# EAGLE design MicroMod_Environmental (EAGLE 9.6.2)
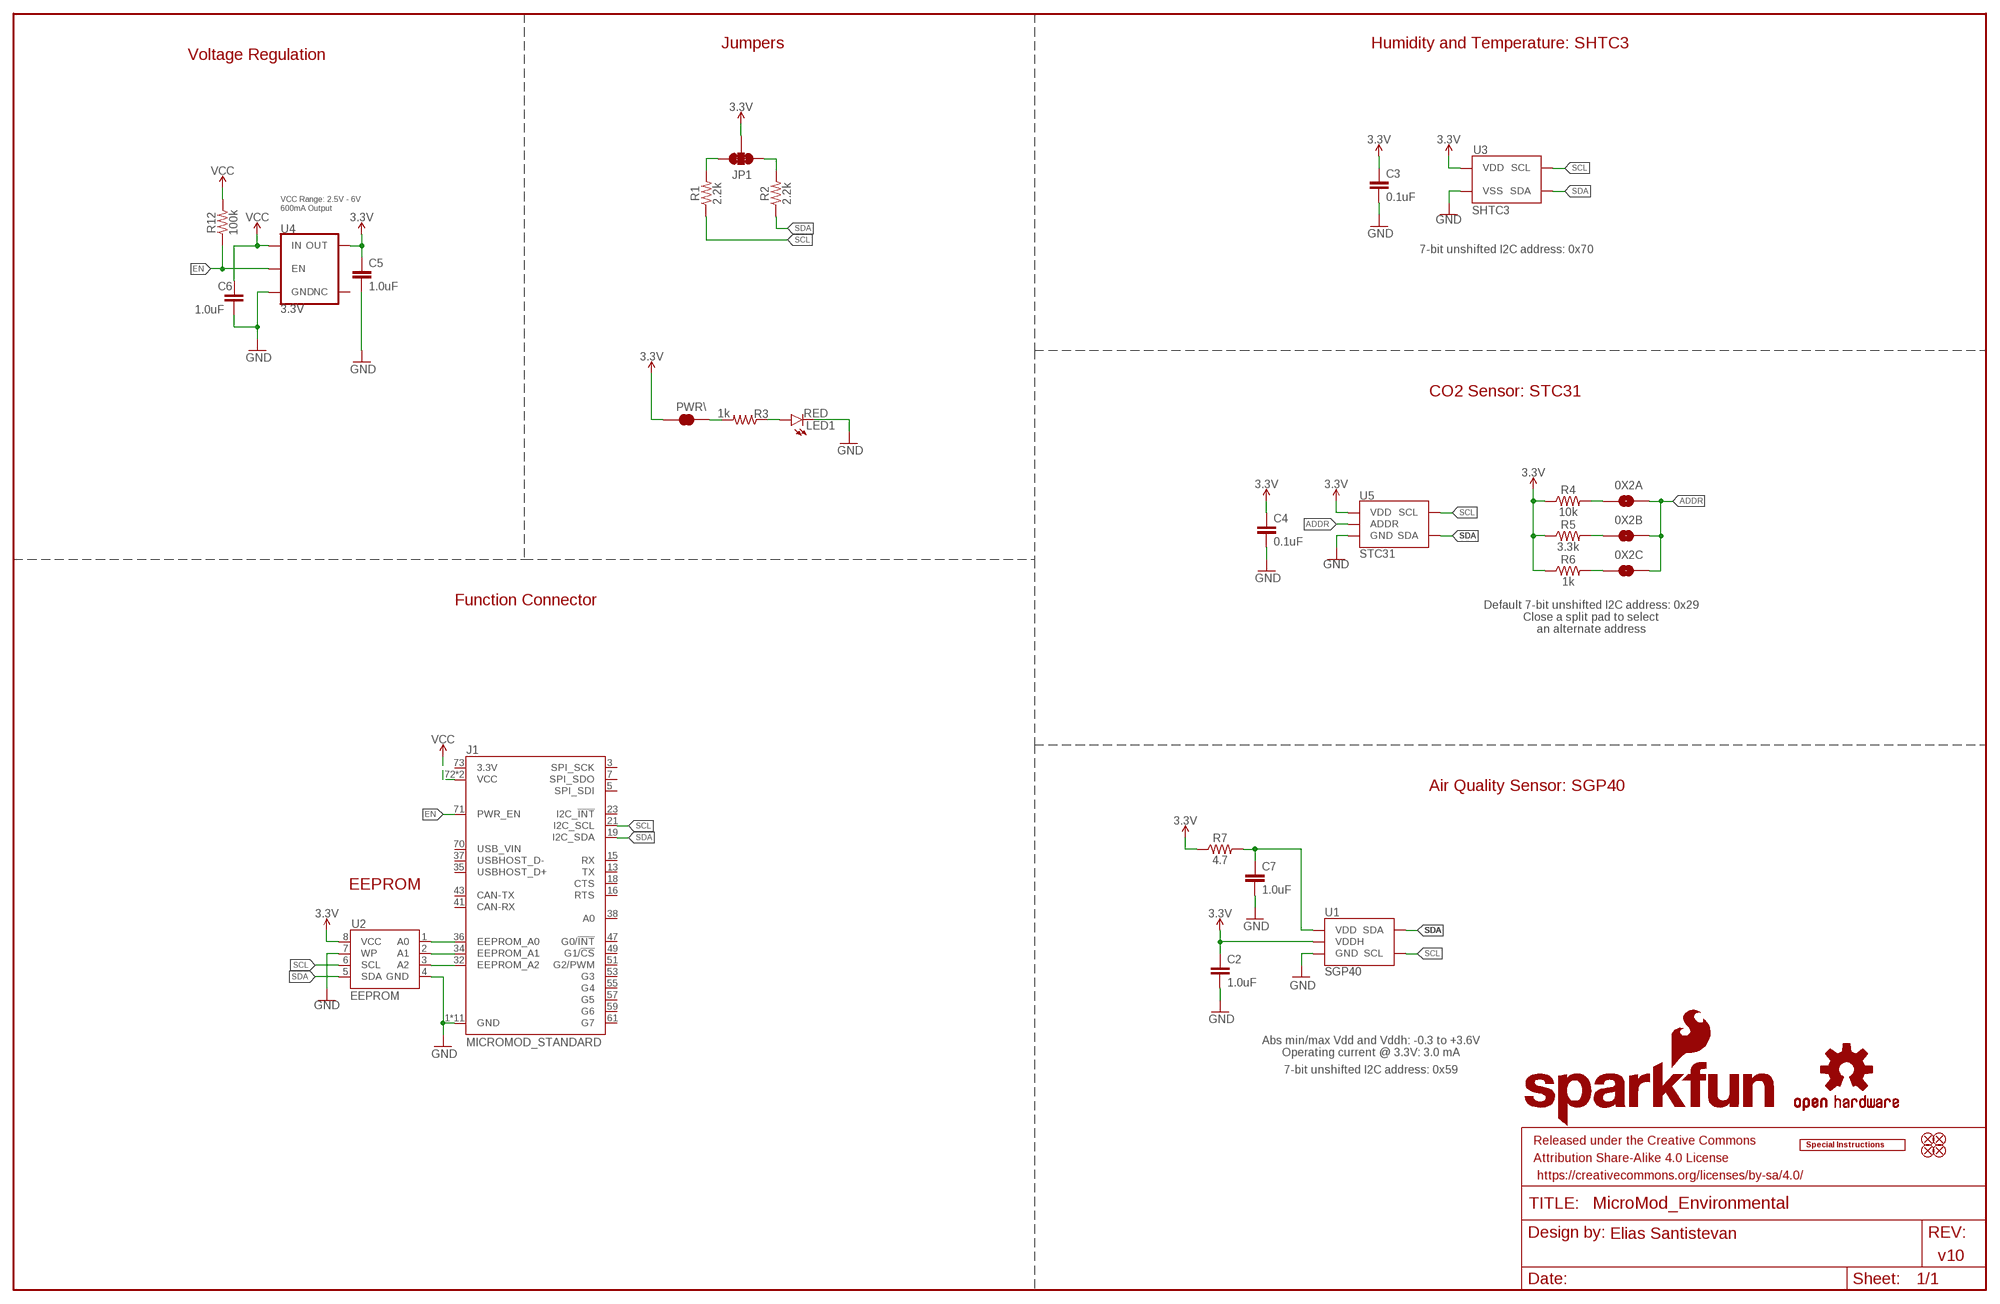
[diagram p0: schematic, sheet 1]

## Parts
0X2A  JUMPER-SMT_2_NO_SILK  [SMT-JUMPER_2_NO_SILK]
0X2B  JUMPER-SMT_2_NO_SILK  [SMT-JUMPER_2_NO_SILK]
0X2C  JUMPER-SMT_2_NO_SILK  [SMT-JUMPER_2_NO_SILK]
C2  1.0uF  1.0UF-0603-16V-10%-X7R  [0603]
C3  0.1uF  0.1UF-0603-25V-5%  [0603]
C4  0.1uF  0.1UF-0603-25V-5%  [0603]
C5  1.0uF  1.0UF-0603-16V-10%  [0603]
C6  1.0uF  1.0UF-0603-16V-10%  [0603]
C7  1.0uF  1.0UF-0603-16V-10%-X7R  [0603]
FD1  FIDUCIAL1X2  [FIDUCIAL-1X2]
FD2  FIDUCIAL1X2  [FIDUCIAL-1X2]
FD3  FIDUCIAL1X2  [FIDUCIAL-1X2]
FD4  FIDUCIAL1X2  [FIDUCIAL-1X2]
FRAME1  FRAME-LEDGER  [CREATIVE_COMMONS]
J1  MICROMOD_STANDARD  [M.2-CARD-E-22_FUNCTION_STANDARD]
JP1  JUMPER-SMT_3_2-NC_TRACE_SILK  [SMT-JUMPER_3_2-NC_TRACE_SILK]
LED1  RED  LED-RED0603  [LED-0603]
LOGO1  SFE_LOGO_NAME_FLAME.2_INCH  [SFE_LOGO_NAME_FLAME_.2]
LOGO2  OSHW-LOGOS  [OSHW-LOGO-S]
LOGO3  SPECIAL_INSTRUCTIONS-ORDERING  [ORDERING_INSTRUCTIONS]
PWR\  JUMPER-SMT_2_NC_TRACE_SILK  [SMT-JUMPER_2_NC_TRACE_SILK]
R1  2.2k  2.2KOHM-0603-1/10W-1%  [0603]
R2  2.2k  2.2KOHM-0603-1/10W-1%  [0603]
R3  1k  1KOHM-0603-1/10W-1%  [0603]
R4  10k  10KOHM-0603-1/10W-1%  [0603]
R5  3.3k  3.3KOHM-0603-1/10W-1%  [0603]
R6  1k  1KOHM-0603-1/10W-1%  [0603]
R7  4.7  4.7OHM-0603-1/10W-1%  [0603]
R12  100k  100KOHM-0603-1/10W-1%  [0603]
U1  SGP40  [SGP40]
U2  EEPROM  EEPROM-I2C512K  [SO08]
U3  SHTC3  [SHTC3]
U4  3.3V  V_REG_AP2112K-3.3V  [SOT23-5]
U5  STC31  [STC31]

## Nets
3.3V [Diff pairs]: C2.1 C3.1 C4.1 C5.1 JP1.2 PWR\.2 R4.1 R5.1 R6.1 R7.1 U1.5(VDDH) U2.8(VCC) U3.1(VDD) U4.5(OUT) U5.6(VDD)
A0: J1.36(EEPROM_A0) U2.1(A0)
A1: J1.34(EEPROM_A1) U2.2(A1)
A2: J1.32(EEPROM_A2) U2.3(A2)
ADDR: 0X2A.2 0X2B.2 0X2C.2 U5.3(ADDR)
EN: J1.71(PWR_EN) R12.1 U4.3(EN)
GND: C2.2 C3.2 C4.2 C5.2 C6.2 C7.2 J1.1(GND) J1.33(GND) J1.39(GND) J1.45(GND) J1.75(GND) J1.GND1(GND) J1.GND2(GND) J1.GND3(GND) J1.GND4(GND) J1.GND5(GND) J1.GND6(GND) LED1.C U1.2(GND) U1.4(GND) U1.DIEPAD(GND) U2.4(GND) U2.7(WP) U3.4(VSS) U3.5(VSS) U4.2(GND) U5.1(GND) U5.5(GND) U5.9(GND) U5.11(GND) U5.DIEPAD(GND)
N$1: PWR\.1 R3.2
N$2: C7.1 R7.2 U1.1(VDD)
N$3: JP1.3 R1.2
N$4: JP1.1 R2.2
N$5: 0X2A.1 R4.2
N$6: 0X2B.1 R5.2
N$7: 0X2C.1 R6.2
N$10: LED1.A R3.1
SCL: J1.21(I2C_SCL) R1.1 U1.6(SCL) U2.6(SCL) U3.2(SCL) U5.4(SCL)
SDA: J1.19(I2C_SDA) R2.1 U1.3(SDA) U2.5(SDA) U3.3(SDA) U5.7(SDA)
VCC: C6.1 J1.72(VCC) J1.74(VCC) R12.2 U4.1(IN)
Unconnected: J1.3(SPI_SCK) J1.5(SPI_SDI) J1.7(SPI_SDO) J1.13(TX) J1.15(RX) J1.16(RTS) J1.18(CTS) J1.23(I2C_!INT!) J1.35(USBHOST_D+) J1.37(USBHOST_D-) J1.38(A0) J1.41(CAN-RX) J1.43(CAN-TX) J1.47(G0/!INT!) J1.49(G1/!CS!) J1.51(G2/PWM) J1.53(G3) J1.55(G4) J1.57(G5) J1.59(G6) J1.61(G7) J1.70(USB_VIN) J1.73(3.3V) U4.4(NC)

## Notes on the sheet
- Jumpers | Humidity and Temperature: SHTC3
- Voltage Regulation
- VCC Range: 2.5V - 6V 
  600mA Output
- 7-bit unshifted I2C address: 0x70
- CO2 Sensor: STC31
- Function Connector
- Default 7-bit unshifted I2C address: 0x29
  Close a split pad to select
  an alternate address
- Air Quality Sensor: SGP40
- EEPROM
- Abs min/max Vdd and Vddh: -0.3 to +3.6V
  Operating current @ 3.3V: 3.0 mA
- 7-bit unshifted I2C address: 0x59
- Elias Santistevan
- v10

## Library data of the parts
0X2A 0X2B 0X2C = SparkFun-Jumpers:JUMPER-SMT_2_NO: Normally open jumper
C2 C7 = SparkFun-Capacitors:1.0UF: 1µF ceramic capacitors; PROD_ID: CAP-13930
C3 C4 = SparkFun-Capacitors:0.1UF: 0.1µF ceramic capacitors; PROD_ID: CAP-08604
C5 C6 = SparkFun-Capacitors:1.0UF: 1µF ceramic capacitors; PROD_ID: CAP-00868
FD1-FD4 = SparkFun-Aesthetics:FIDUCIAL: Fiducial Alignment Points
FRAME1 = SparkFun-Aesthetics:FRAME-LEDGER: Schematic Frame - Ledger
J1 = SparkFun-MicroMod-Function:MICROMOD: MicroMod Connector Description: A card edge connector and mating PCB connector to allow various MicroMod Processor Boards to be coupled with various carrier boards of different capabilities. Based on the M.2 standard.
JP1 = SparkFun-Jumpers:JUMPER-SMT_3_2-NC_TRACE: Normally closed trace jumper (2 of 2 connections) This jumper has a trace between all three pads so they are normally closed (NC). Use a razor knife to open the connection(s). For best results follow the IPC guidelines for cutting traces: Cutout at least 0.063 mm (0.005 in). Remove all loose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
LED1 = SparkFun-LED:LED-RED: Red SMD LED; PROD_ID: DIO-00819
LOGO1 = SparkFun-Aesthetics:SFE_LOGO_NAME_FLAME: SparkFun Font Logo w/ Flame
LOGO2 = SparkFun-Aesthetics:OSHW-LOGO: Open-Source Hardware (OSHW) Logo
LOGO3 = SparkFun-Aesthetics:SPECIAL_INSTRUCTIONS: Special Ordering/Production Instructions Alert
PWR\ = SparkFun-Jumpers:JUMPER-SMT_2_NC_TRACE: Normally closed trace jumper
R1 R2 = SparkFun-Resistors:2.2KOHM: 2.2kΩ resistor; PROD_ID: RES-08272
R3 R6 = SparkFun-Resistors:1KOHM: 1kΩ resistor; PROD_ID: RES-07856
R4 = SparkFun-Resistors:10KOHM: 10kΩ resistor; PROD_ID: RES-00824
R5 = SparkFun-Resistors:3.3KOHM: 3.3kΩ resistor; PROD_ID: RES-07851
R7 = SparkFun-Resistors:4.7OHM: 4.7Ω resistor; PROD_ID: RES-15581
R12 = SparkFun-Resistors:100KOHM: 100kΩ resistor; PROD_ID: RES-07828
U1 = SparkFun-Sensors:SGP40: The SGP40 is a digital gas sensor designed for easy integration into air purifiers or demand-controlled ventilation systems.; DIGIKEY_PART: 1649-SGP40-D-R4CT-ND; PROD_ID: IC-15580
U2 = SparkFun-IC-Memory:EEPROM-I2C: I2C EEPROMs, 24LC256 and others 24LC256 Series 256 kb I2C 2 Wire (32 k x 8 Bit) 2.5 V Serial EEPROM SMD - SOIC-8 Datasheet SparkFun Products SparkFun UDB5 - PIC UAV Development Board (GPS-11703); PROD_ID: IC-14645
U3 = SparkFun-Sensors:SHTC3: Sensirion SHTC3 Humidity Sensor The SHTC3 is a digital humidity and temperature sensor designed especially for battery-driven high-volume consumer electronics applications.; PROD_ID: IC-14840
U4 = SparkFun-IC-Power:V_REG_AP2112: AP2112 - 600mA CMOS LDO Regulator w/ Enable The AP2112 is CMOS process low dropout linear regulator with enable function, the regulator delivers a guaranteed 600mA (min.) continuous load current. Features Output Voltage Accuracy: ±1.5% Output Current: 600mA (Min.) Foldback Short Current Protection: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; PROD_ID: VREG-12457
U5 = SparkFun-Sensors:STC31: STC31 CO2 Sensor Based on Thermal Conductivity; MANU_PART: STC31-R3; PROD_ID: IC-16076

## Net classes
1 Antenna: width 1 mm, clearance 0.3 mm

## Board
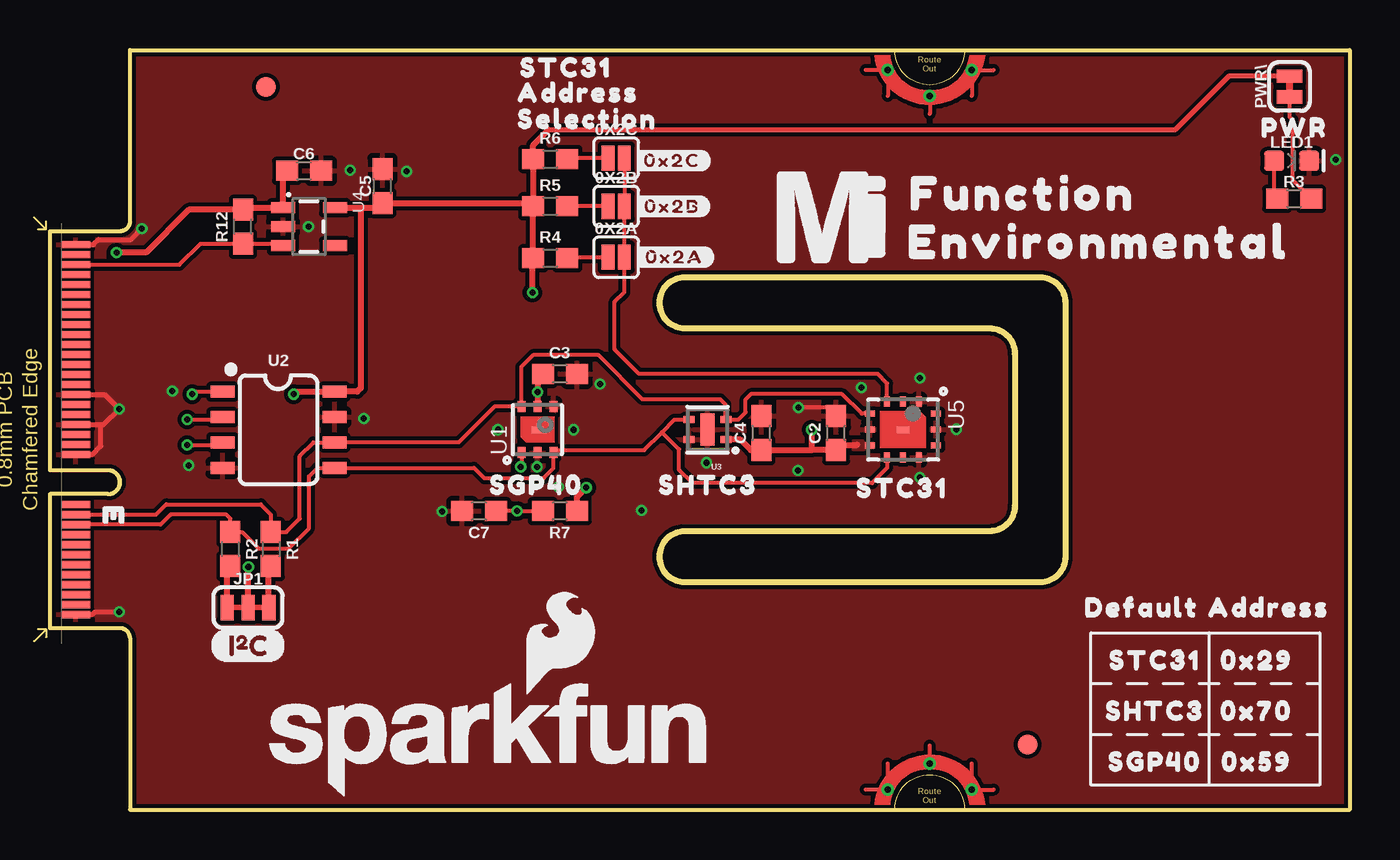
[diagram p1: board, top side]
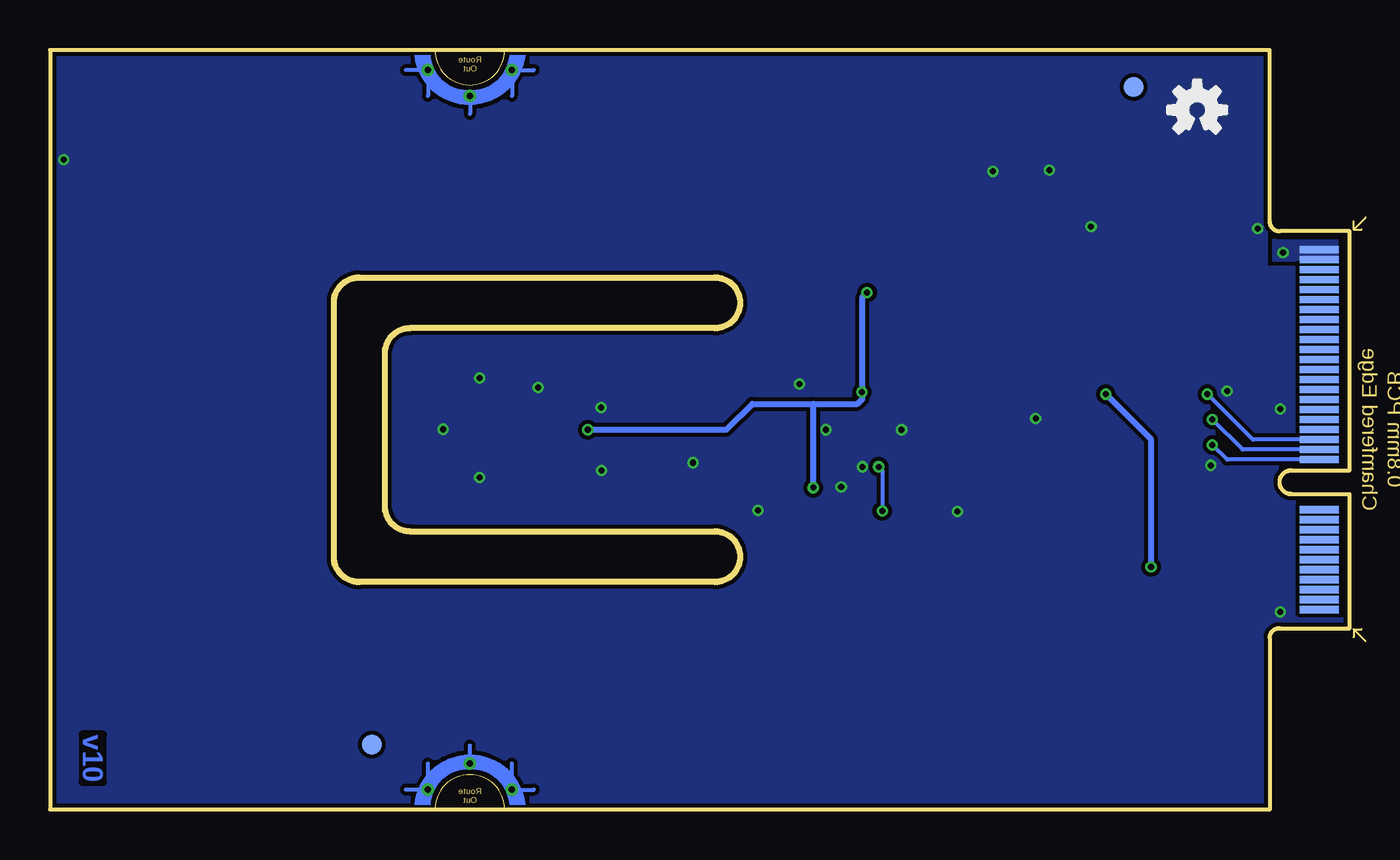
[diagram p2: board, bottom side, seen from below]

Size 65 x 38 mm. Coordinates in mm from the lower left corner, seen from the top.
Outline: 0,9.07 0,15.77 2.9,15.77 arc180 2.9,16.97 0,16.97 0,28.93 3.5,28.93 arc84 4,29.4 4,38 65,38 65,0 4,0 4,8.6 arc85 3.5,9.07 0,9.07
Outline: 30.48,12.65 arc90 31.75,11.38 49.53,11.38 arc90 50.8,12.65 50.8,25.35 arc90 49.53,26.62 31.75,26.62 arc90 30.48,25.35 arc90 31.75,24.08 46.99,24.08 arc-90 48.26,22.81 48.26,15.19 arc-90 46.99,13.92 31.75,13.92 arc90 30.48,12.65
Copper layers (1*16): Top 0.035mm / dielectric 1.5mm / Bottom 0.035mm
Design rules "SparkFun-2-Layer-Minimum-JLCPCB": minimum track width 5mil, minimum drill 0.3mm, track to track 5mil, track to pad 5mil, pad to pad 5mil, via to via 5mil, smd to smd 5mil, copper to edge 7mil, drill to drill 7mil, minimum pad ring 5mil, minimum via ring 5mil, stop-mask expansion 2.5mil, vias tented up to drill 25mil, thermal gap 10mil

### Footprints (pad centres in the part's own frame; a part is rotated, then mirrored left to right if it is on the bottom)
SMT-JUMPER_2_NO_SILK = smd 0.635 x 1.27: 1 -0.406,0; 2 0.406,0
0603 = smd 1.1 x 1: 1 -0.85,0; 2 0.85,0
FIDUCIAL-1X2 = smd 1 x 1: 1 0,0
M.2-CARD-E-22_FUNCTION_STANDARD = smd 0.35 x 1.45: 1 9.25,1.275; 3 8.75,1.275; 5 8.25,1.275; 7 7.75,1.275; 9 7.25,1.275; 11 6.75,1.275; 13 6.25,1.275; 15 5.75,1.275; 17 5.25,1.275; 19 4.75,1.275; 21 4.25,1.275; 23 3.75,1.275; 33 1.25,1.275; 35 0.75,1.275; 37 0.25,1.275; 39 -0.25,1.275; 41 -0.75,1.275; 43 -1.25,1.275; 45 -1.75,1.275; 47 -2.25,1.275; 49 -2.75,1.275; 51 -3.25,1.275; 53 -3.75,1.275; 55 -4.25,1.275; 57 -4.75,1.275; 59 -5.25,1.275; 61 -5.75,1.275; 63 -6.25,1.275; 65 -6.75,1.275; 67 -7.25,1.275; 69 -7.75,1.275; 71 -8.25,1.275; 73 -8.75,1.275; 75 -9.25,1.275 | smd 0.35 x 1.95 bottom: 2 9,1.525; 4 8.5,1.525; 6 8,1.525; 8 7.5,1.525; 10 7,1.525; 12 6.5,1.525; 14 6,1.525; 16 5.5,1.525; 18 5,1.525; 20 4.5,1.525; 22 4,1.525; 32 1.5,1.525; 34 1,1.525; 36 0.5,1.525; 38 0,1.525; 40 -0.5,1.525; 42 -1,1.525; 44 -1.5,1.525; 46 -2,1.525; 48 -2.5,1.525; 50 -3,1.525; 52 -3.5,1.525; 54 -4,1.525; 56 -4.5,1.525; 58 -5,1.525; 60 -5.5,1.525; 62 -6,1.525; 64 -6.5,1.525; 66 -7,1.525; 68 -7.5,1.525; 70 -8,1.525; 72 -8.5,1.525; 74 -9,1.525 | drill 0.305 pad 0.61: GND1 -18,41.9; GND2 -16.7,44; GND3 -18,46.1; GND4 18,41.9; GND5 16.7,44; GND6 18,46.1
SMT-JUMPER_3_2-NC_TRACE_SILK = smd 0.66 x 1.27: 1 -1.041,0; 2 0,0; 3 1.041,0
LED-0603 = smd 1 x 1: A -0.877,0; C 0.877,0
SMT-JUMPER_2_NC_TRACE_SILK = smd 0.66 x 1.27: 1 -0.521,0; 2 0.521,0
SGP40 = smd 0.55 x 0.4: 1 -1.15,0.8; 2 -1.15,0; 3 -1.15,-0.8; 4 1.15,-0.8; 5 1.15,0; 6 1.15,0.8 | smd 0.305 x 0.61: DIEPAD 0,0
SO08 = smd 0.6 x 1.2: 1 -1.905,-2.8; 2 -0.635,-2.8; 3 0.635,-2.8; 4 1.905,-2.8; 5 1.905,2.8; 6 0.635,2.8; 7 -0.635,2.8; 8 -1.905,2.8
SHTC3 = smd 0.55 x 0.35: 1 -0.925,0.5; 2 -0.925,-0.5; 3 0.925,-0.5; 4 0.925,0.5 | smd 0.7 x 1.6: 5 0,0
SOT23-5 = smd 0.55 x 1.2: 1 -0.95,-1.3; 2 0,-1.3; 3 0.95,-1.3; 4 0.95,1.3; 5 -0.95,1.3
STC31 = smd 0.5 x 0.3: 1 -1.4,0.8; 2 -1.4,0; 3 -1.4,-0.8; 7 1.4,-0.8; 8 1.4,0; 9 1.4,0.8 | smd 0.3 x 0.5: 4 -0.8,-1.65; 5 0,-1.65; 6 0.8,-1.65; 10 0.8,1.65; 11 0,1.65; 12 -0.8,1.65 | smd 0.305 x 0.61: DIEPAD 0,0

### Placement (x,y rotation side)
0X2A  28.32,27.64 0 top
0X2B  28.32,30.18 0 top
0X2C  28.32,32.59 0 top
C2  39.32,18.83 90 top
C3  25.5,21.79 0 top
C4  35.59,18.83 90 top
C5  16.64,31.19 90 top
C6  12.7,31.95 0 top
C7  21.46,14.94 180 top
FD1  10.79,36.15 0 top
FD2  10.79,36.15 0 bottom
FD3  48.9,3.25 0 bottom
FD4  48.9,3.25 0 top
FRAME1  not placed on the board
J1  0,19 270 top
JP1  9.91,10.11 0 top
LED1  62.1,32.46 0 top
LOGO1  21.97,3.51 0 top
LOGO2  7.62,35 0 bottom
LOGO3  not placed on the board
PWR\  62,36.17 90 top
R1  11.05,13.03 270 top
R2  9.02,13.03 270 top
R3  62.23,30.56 0 top
R4  25.02,27.59 0 top
R5  25.02,30.18 0 top
R6  25.02,32.54 0 top
R7  25.5,14.94 180 top
R12  9.65,29.16 90 top
U1  24.38,19 90 top
U2  11.43,19 270 top
U3  32.89,19 180 top
U4  12.95,29.16 270 top
U5  42.67,19 270 top
U$1  [#0X2A#21]  31.24,27.64 0 top
U$2  [#0X2B#21]  31.11,30.18 0 top
U$3  [#0X2C#21]  31.11,32.46 0 top
U$4  [PWR321541]  62.23,34.11 0 top
U$5  [FUNCTION524]  48.64,30.81 0 top
U$6  [ENVIRONMENTAL526]  52.45,28.4 0 top
U$7  [MICROMOD_MI_LOGO_1]  39.12,29.67 0 top
U$8  [I2C]  8,8.21 0 top
U$9  [ADDRESS40313505]  26.42,35.87 0 top
U$10  [0X2940313520]  60.35,7.47 0 top
U$11  [SGP40313503]  24.33,16.23 0 top
U$12  [SHTC3501]  32.92,16.23 0 top
U$13  [STC313502]  25.81,37.11 0 top
U$14  [DEFAULT40313504]  54.61,10.11 0 top
U$15  [ADDRESS40313505]  60.96,10.11 0 top
U$16  [STC313502]  55.27,7.47 0 top
U$17  [SHTC3501]  55.27,4.93 0 top
U$18  [SGP40313503]  55.27,2.39 0 top
U$19  [0X5940313520]  60.35,2.39 0 top
U$20  [0X7040313520]  60.35,4.93 0 top
U$21  [SELECTION40313506]  26.87,34.54 0 top
U$22  [STC313502]  42.62,16.08 0 top

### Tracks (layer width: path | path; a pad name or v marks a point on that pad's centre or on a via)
3.3V  (via drill 0.3)
  Top 0.254: 24.94,34.01 56.29,34.01 58.97,36.69 PWR\.2
  Top 0.305: U4.5 15.54,30.11 | 15.54,30.11 16.41,30.11 C5.1 24,30.34 24.02,30.32 | v24.13,25.86 24.13,27.55 R4.1 R5.1 24.02,30.32 | 15.54,30.11 15.54,21.08 15.37,20.9 U2.8 12.32,20.9 v12.19,20.78 | C3.1 24.38,21.53 v24.38,20.88 U1.5 | 40.39,18.24 39.57,18.24 C2.1 38.1,17.98 | 38.1,17.98 38.1,17.97 C4.1 35.05,17.98 34.54,18.5 U3.1 | 38.1,17.98 v38.1,19 | JP1.2 9.91,12.12 v9.92,12.14 | R7.1 26.35,15.63 v26.82,16.1 | 24.94,34.01 24.17,33.24 R6.1 24.17,30.47 24.02,30.32
  Bottom 0.305: 26.82,20.29 29.87,20.29 31.17,19 v38.1,19 | 26.82,20.29 24.61,20.29 24.38,20.52 v24.38,20.88 24.38,25.6 v24.13,25.86 | v9.92,12.14 9.92,18.51 v12.19,20.78 | v26.82,16.1 26.82,20.29
  pour Top (isolate 0.305, no thermals): 41.17,18.34 40.79,18.34 40.67,18.47 40.16,18.47 40.16,17.98 40.72,17.98 40.82,18.09 41.17,18.09
A0  (via drill 0.3)
  Top 0.203: v7.11,20.78 7.24,20.9 U2.1
  Bottom 0.203: J1.36 4.83,18.5 v7.11,20.78
A1  (via drill 0.3)
  Top 0.203: v6.86,19.51 8.5,19.51 U2.2
  Bottom 0.203: J1.34 5.35,18 v6.86,19.51
A2  (via drill 0.3)
  Top 0.203: v6.86,18.24 8.5,18.24 U2.3
  Bottom 0.203: J1.32 6.12,17.5 v6.86,18.24
ADDR
  Top 0.203: 0X2C.2 0X2B.2 0X2A.2 28.73,25.88 28.25,25.4 28.25,23.01 29.46,21.79 41.4,21.79 41.87,21.32 U5.3
EN
  Top 0.203: J1.71 6.47,27.25 7.53,28.31 R12.1 11.55,28.31 U4.3
GND  (via drill 0.3)
  Top 0.203: J1.GND4 43.2,2.3 J1.GND5 44.8,2.3 J1.GND6 | J1.GND1 43.2,35.7 J1.GND2 44.03,35.73 44.93,35.73 46.1,36.9 J1.GND3 | C2.2 38.89,20.12 v37.44,20.12
  Top 0.254: J1.39 2.54,19.25 | 2.54,19.25 2.66,19.25 v3.45,20.04 2.75,20.75 J1.45 | J1.33 1.29,17.77 2.13,17.77 2.54,18.18 2.54,19.25 | J1.75 2.16,28.25 2.43,28.51 4.05,28.51 v4.6,29.06 | J1.1 1.29,9.77 2.13,9.77 2.24,9.88 v3.45,9.88
  other vias: 19.61,14.91 64.31,32.51 6.93,17.22 15.7,19.56 17.83,31.93 15.01,31.98 12.93,29.16 29.59,14.96 27.51,21.29 45.34,19.03 43.51,16.61 32.84,17.35 25.43,16.13 26.19,19 22.4,19 43.51,21.59 24.36,17.15 40.59,21.11 37.41,16.97 6.12,20.93
  pour Bottom (isolate 0.203, rank 4): 0,38.05 65.02,38.05 65.02,-0.05 0,-0.05
  pour Top (isolate 0.203, rank 4): 0,38.05 65.02,38.05 65.02,-0.05 0,-0.05
N$1
  Top 0.203: R3.2 62.15,31.48 62.15,34.49 62,34.65 PWR\.1
N$2  (via drill 0.3)
  Top 0.203: U1.1 23.58,17.18 v23.55,17.15 | R7.2 v23.37,14.94 C7.1
  Bottom 0.203: v23.55,17.15 23.37,16.97 v23.37,14.94
N$3
  Top 0.305: JP1.3 10.95,12.08 R1.2
N$4
  Top 0.305: JP1.1 8.87,12.03 R2.2
N$5
  Top 0.203: R4.2 25.92,27.64 0X2A.1
N$6
  Top 0.203: 0X2B.1 R5.2
N$7
  Top 0.203: 0X2C.1 25.92,32.59 R6.2
N$10
  Top 0.203: R3.1 61.23,30.71 LED1.A
SCL
  Top 0.203: J1.21 5.31,14.75 5.83,15.27 10.54,15.27 11.05,14.76 R1.1 11.82,13.88 12.5,14.55 12.5,17.68 13.18,18.36 U2.6 20.45,18.36 22.23,20.15 U1.6 23.58,22.15 24.19,22.76 27.41,22.76 29.64,20.52 33.53,20.52 33.78,20.27 33.78,19.54 U3.2 34.43,19.5 34.8,19.86 34.8,20.52 35.05,20.78 39.62,20.78 40.6,19.8 U5.4
SDA
  Top 0.203: J1.19 5.54,14.25 6.05,14.76 8.81,14.76 9.02,14.55 R2.1 9.6,13.88 10.43,13.05 11.94,13.05 12.95,14.07 12.95,16.66 13.39,17.09 U2.5 21.21,17.09 21.72,16.59 24.69,16.59 25.18,17.08 U1.3 25.32,17.98 29.72,17.98 30.61,18.87 | 30.61,18.87 31.23,19.5 U3.3 | U5.7 41.87,17.09 41.11,16.33 32.13,16.33 31.46,17 31.46,18.02 30.61,18.87
VCC  (via drill 0.3)
  Top 0.305: v3.33,27.86 4.8,27.86 6.95,30.01 R12.2 9.75,30.11 U4.1 11.65,31.76 C6.1
  pour Bottom (isolate 0.305, no thermals): 0.61,28.55 3.81,28.55 3.81,27.46 0.61,27.46

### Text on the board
Bottom: v10
tDocu: ENIG Finish | 0.8mm PCB | Chamfered Edge | Elias Santistevan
